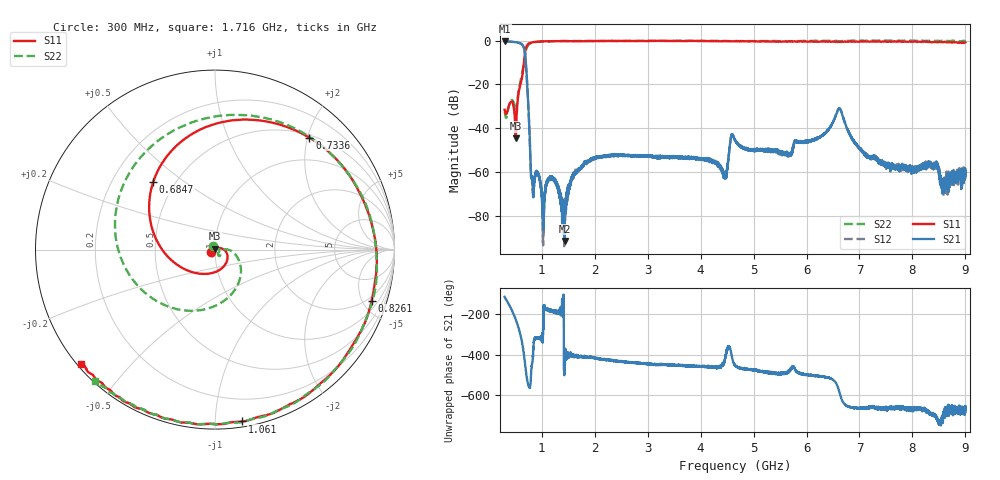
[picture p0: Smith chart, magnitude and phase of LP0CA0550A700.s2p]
!Agilent Technologies,E8358A,US41080443,A.07.50.56
!Agilent E8358A: A.07.50.56
!Date: Monday, December 14, 2015 12:33:17
!Correction: S11(Full 2 Port(1,2))
!S21(Full 2 Port(1,2))
!S12(Full 2 Port(1,2))
!S22(Full 2 Port(1,2))
!S2P File: Measurements: S11, S21, S12, S22:
# Hz S  dB  R 50
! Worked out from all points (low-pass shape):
!   6401 points, 300 MHz to 9 GHz, reference 50 ohm
!   highest |S21| = -0.30 dB at 300 MHz (marker M1); lowest = -91.6 dB at 1.431 GHz (marker M2)
!   |S21| within 3 dB of the highest: start of sweep to 663.8 MHz
!   lowest |S11| = -44.7 dB at 509.3 MHz (marker M3), VSWR 1.01, Z = 49.7 + j0.519 ohm
!   |S11| at or under -10 dB: start of sweep to 664.7 MHz
!   |S22| runs from -35.3 to 0.1 dB; largest |S21 - S12| = 0.0066
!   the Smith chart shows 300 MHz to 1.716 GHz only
!   S11 on the Smith chart (normalised r, x): 300 MHz: 0.95, -0.02; 684.7 MHz: 0.38, +0.39; 733.6 MHz: 0.54, +2.03; 826.1 MHz: 1.58, -5.80; 1.061 GHz: 0.04, -1.17; 1.716 GHz: 0.01, -0.37
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3e8  -31.56 -155.1  -0.30 -114.6  -0.30 -114.3  -32.41 111.2
4.223438e8  -27.86 -116.4  -0.47 -172.8  -0.46 -172.6  -27.40 -46.0
5.093438e8  -44.71 116.3  -0.68 134.7  -0.67 134.9  -32.09 -37.7
6.194531e8  -17.90 -92.1  -1.53 34.4  -1.52 34.7  -16.31 -26.7
6.847031e8  -5.85 132.5  -6.13 -82.0  -6.12 -81.7  -6.68 -150.5
7.336406e8  -1.77 49.9  -23.00 -174.9  -22.99 -174.4  -2.50 85.8
8.260781e8  -0.74 -18.3  -65.63 -74.0  -65.76 -69.5  -0.88 -4.0
1.06125e9  -0.27 -81.1  -68.75 -174.4  -70.52 -161.1  -0.28 -74.0
1.203984e9  -0.19 -100.1  -63.04 173.4  -62.82 176.2  -0.23 -93.8
1.431e9  -0.13 -120.4  -91.58 -107.3  -76.93 -91.0  -0.19 -115.1
1.716469e9  -0.18 -139.6  -58.45 -47.1  -58.77 -49.8  -0.10 -132.4
1.750453e9  -0.23 -141.3  -57.90 -49.0  -57.49 -49.8  -0.12 -134.3
3.200906e9  -0.04 -176.9  -53.25 -87.1  -53.37 -86.7  -0.16 -172.3
4.458328e9  -0.26 169.9  -61.22 -62.9  -63.02 -61.2  -0.10 164.0
4.65e9  -0.21 168.5  -45.27 -89.9  -45.28 -91.5  -0.17 159.4
6.100453e9  -0.30 142.9  -45.47 -138.9  -45.67 -138.9  -0.10 126.0
6.623812e9  -0.58 137.0  -30.97 133.0  -30.92 135.0  -0.26 127.1
6.999e9  -0.37 137.3  -49.00 55.7  -48.92 59.9  0.01 130.6
7.550906e9  -0.35 141.2  -56.87 58.7  -57.23 57.6  0.01 134.0
8.435859e9  -0.56 145.4  -57.48 14.2  -55.50 15.9  -0.14 128.8
8.590828e9  -0.60 144.0  -62.79 31.2  -64.98 22.6  -0.01 127.1
9e9  -0.71 139.8  -59.54 66.6  -63.31 61.7  -0.19 118.3
